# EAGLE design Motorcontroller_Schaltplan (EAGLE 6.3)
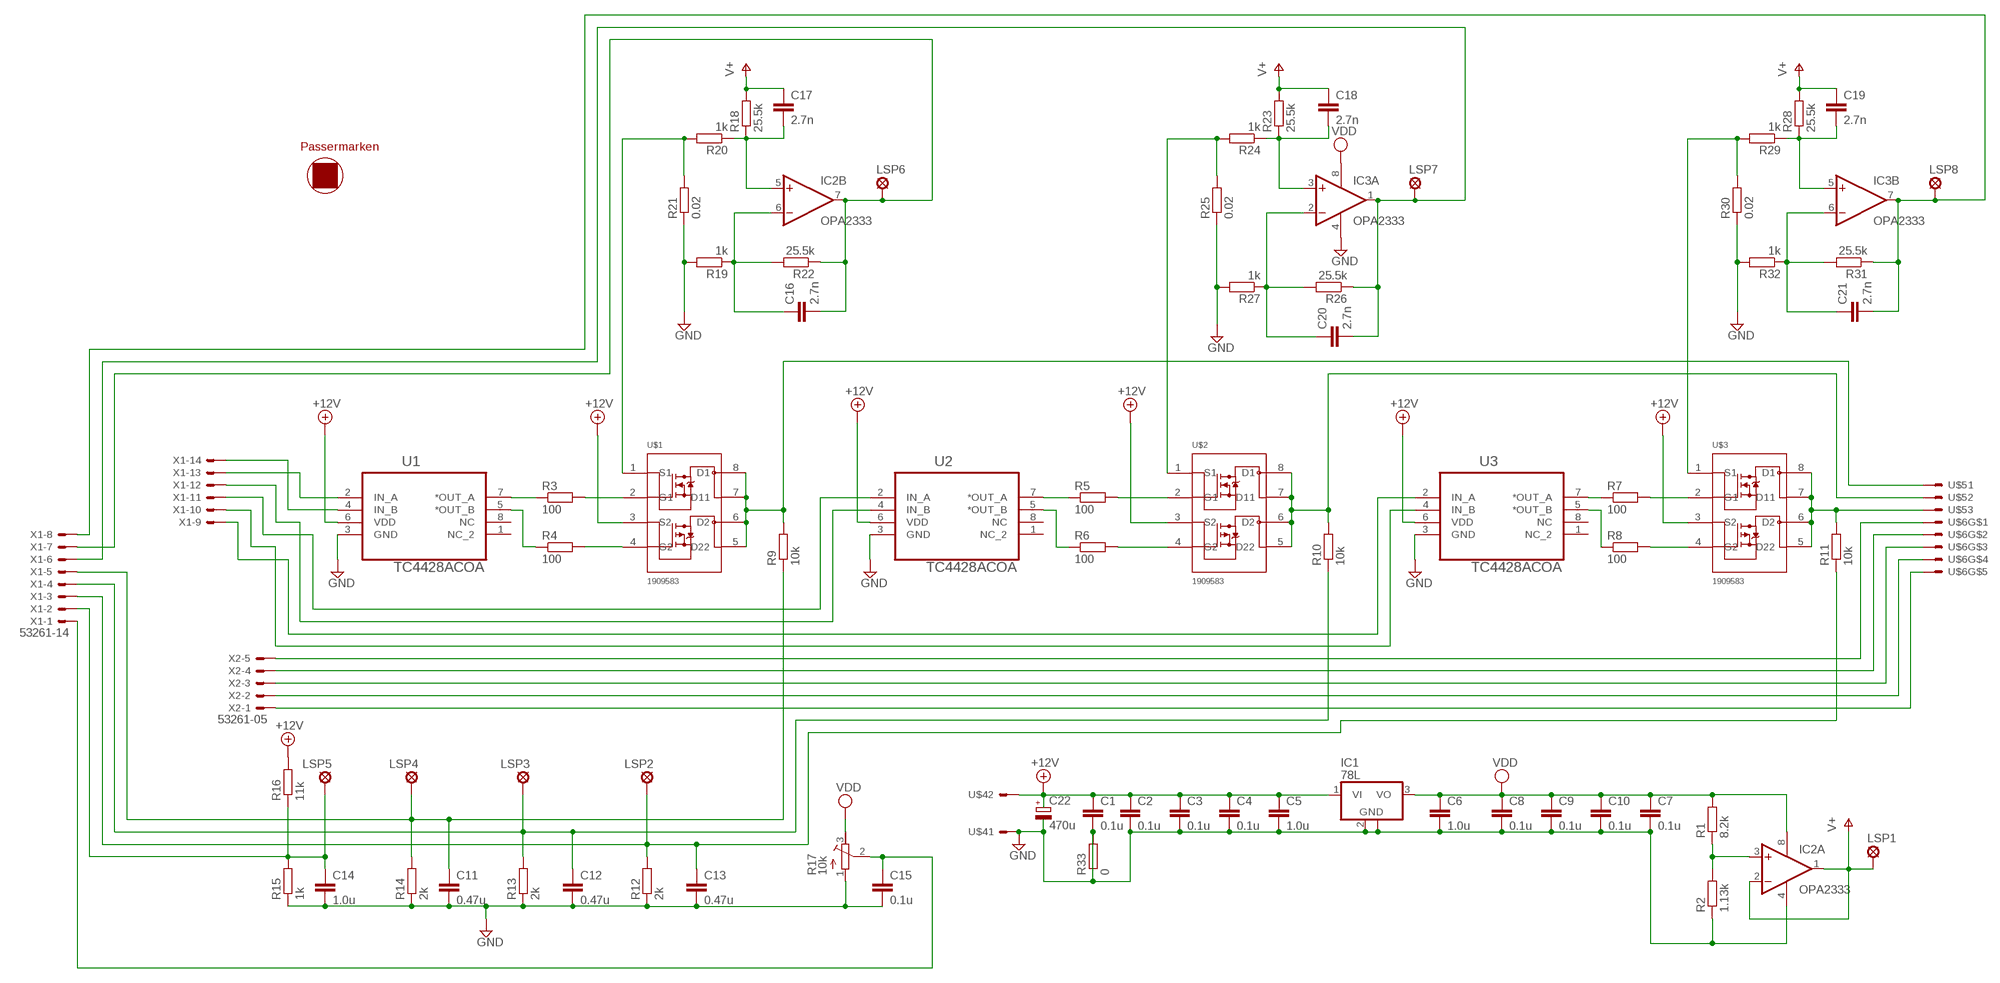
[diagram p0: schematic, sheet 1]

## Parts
C1  0.1u  C-EUC0603  [C0603]
C2  0.1u  C-EUC0603  [C0603]
C3  0.1u  C-EUC0603  [C0603]
C4  0.1u  C-EUC0603  [C0603]
C5  1.0u  C-EUC0603  [C0603]
C6  1.0u  C-EUC0603  [C0603]
C7  0.1u  C-EUC0603  [C0603]
C8  0.1u  C-EUC0603  [C0603]
C9  0.1u  C-EUC0603  [C0603]
C10  0.1u  C-EUC0603  [C0603]
C11  0.47u  C-EUC0603  [C0603]
C12  0.47u  C-EUC0603  [C0603]
C13  0.47u  C-EUC0603  [C0603]
C14  1.0u  C-EUC0603  [C0603]
C15  0.1u  C-EUC0603  [C0603]
C16  2.7n  C-EUC0603  [C0603]
C17  2.7n  C-EUC0603  [C0603]
C18  2.7n  C-EUC0603  [C0603]
C19  2.7n  C-EUC0603  [C0603]
C20  2.7n  C-EUC0603  [C0603]
C21  2.7n  C-EUC0603  [C0603]
C22  470u  CPOL-EU150CLZ-1010  [150CLZ-1010]
IC1  78L  [SOT223]
IC2  OPA2333  [SOIC8]
IC3  OPA2333  [SOIC8]
LSP1  MCS10B  [MCS10B]
LSP2  MCS10B  [MCS10B]
LSP3  MCS10B  [MCS10B]
LSP4  MCS10B  [MCS10B]
LSP5  MCS10B  [MCS10B]
LSP6  MCS10B  [MCS10B]
LSP7  MCS10B  [MCS10B]
LSP8  MCS10B  [MCS10B]
R1  8.2k  R-EU_R0603  [R0603]
R2  1.13k  R-EU_R0603  [R0603]
R3  100  R-EU_R0603  [R0603]
R4  100  R-EU_R0603  [R0603]
R5  100  R-EU_R0603  [R0603]
R6  100  R-EU_R0603  [R0603]
R7  100  R-EU_R0603  [R0603]
R8  100  R-EU_R0603  [R0603]
R9  10k  R-EU_R0603  [R0603]
R10  10k  R-EU_R0603  [R0603]
R11  10k  R-EU_R0603  [R0603]
R12  2k  R-EU_R0603  [R0603]
R13  2k  R-EU_R0603  [R0603]
R14  2k  R-EU_R0603  [R0603]
R15  1k  R-EU_R0603  [R0603]
R16  11k  R-EU_R0603  [R0603]
R17  10k  R-TRIMM  [TRIMMER3150]
R18  25.5k  R-EU_R0603  [R0603]
R19  1k  R-EU_R0603  [R0603]
R20  1k  R-EU_R0603  [R0603]
R21  0.02  R-EU_R1206  [R1206]
R22  25.5k  R-EU_R0603  [R0603]
R23  25.5k  R-EU_R0603  [R0603]
R24  1k  R-EU_R0603  [R0603]
R25  0.02  R-EU_R1206  [R1206]
R26  25.5k  R-EU_R0603  [R0603]
R27  1k  R-EU_R0603  [R0603]
R28  25.5k  R-EU_R0603  [R0603]
R29  1k  R-EU_R0603  [R0603]
R30  0.02  R-EU_R1206  [R1206]
R31  25.5k  R-EU_R0603  [R0603]
R32  1k  R-EU_R0603  [R0603]
R33  0  R-EU_R2010  [R2010]
U1  TC4428ACOA  [SOIC127P600X175-8N]
U2  TC4428ACOA  [SOIC127P600X175-8N]
U3  TC4428ACOA  [SOIC127P600X175-8N]
U$1  1909583  [SO8]
U$2  1909583  [SO8]
U$3  1909583  [SO8]
U$4  PTSM0.5/3-2.5-HSMDR44  [PTSM0,5/2-2,5-HSMDR44]
U$5  PTSM0.5/3-2.5-HSMDR44  [PTSM0,5/3-2,5-HSMDR44]
U$6  PTSM0.5/5-2.5-HSMDR44  [PTSM0,5/5-2,5-HSMDR44]
U$7  PASSERMARKEN  [MASTERSUBSTRAT-MITPASSERMARKEN]
X1  53261-14  [53261-14]
X2  53261-05  [53261-05]

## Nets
+12V: C1.1 C2.1 C3.1 C4.1 C5.1 C22.+ IC1.1(VI) R16.2 U1.6(VDD) U2.6(VDD) U3.6(VDD) U$1.3(S2) U$2.3(S2) U$3.3(S2) U$4.2
GND: C1.2 C2.2 C3.2 C4.2 C5.2 C6.2 C7.2 C8.2 C9.2 C10.2 C11.2 C12.2 C13.2 C14.2 C15.2 C22.- IC1.2(GND) IC1.4(GND) IC2.4(P:V-) IC3.4(P:V-) R2.1 R12.1 R13.1 R14.1 R15.1 R17.1 R19.2 R21.1 R25.1 R27.2 R30.1 R32.2 R33.1 R33.2 U1.3(GND) U2.3(GND) U3.3(GND) U$4.1
N$1: U1.4(IN_B) X1.14
N$2: IC2.3(A:+IN) R1.1 R2.2
N$3: U1.2(IN_A) X1.13
N$4: R3.1 U1.7(*OUT_A)
N$5: R3.2 U$1.2(G1)
N$6: R4.1 U1.5(*OUT_B)
N$7: R4.2 U$1.4(G2)
N$8: R9.2 U$1.5(D22) U$1.6(D2) U$1.7(D11) U$1.8(D1) U$5.1
N$9: U$6.1 X2.5
N$11: U2.4(IN_B) X1.12
N$12: R5.1 U2.7(*OUT_A)
N$13: R6.1 U2.5(*OUT_B)
N$14: R5.2 U$2.2(G1)
N$15: R6.2 U$2.4(G2)
N$16: R10.2 U$2.5(D22) U$2.6(D2) U$2.7(D11) U$2.8(D1) U$5.2
N$17: U2.2(IN_A) X1.11
N$18: U3.4(IN_B) X1.10
N$19: R7.1 U3.7(*OUT_A)
N$20: R7.2 U$3.2(G1)
N$21: R8.1 U3.5(*OUT_B)
N$22: R8.2 U$3.4(G2)
N$23: R11.2 U$3.5(D22) U$3.6(D2) U$3.7(D11) U$3.8(D1) U$5.3
N$24: U$6.2 X2.4
N$25: C13.1 LSP2.MP R11.1 R12.2 X1.3
N$26: U3.2(IN_A) X1.9
N$28: C11.1 LSP4.MP R9.1 R14.2 X1.5
N$29: C12.1 LSP3.MP R10.1 R13.2 X1.4
N$31: C14.1 LSP5.MP R15.2 R16.1 X1.2
N$32: C15.1 R17.2 X1.1
N$33: C18.2 IC3.3(A:+IN) R23.1 R24.1
N$34: C17.2 IC2.5(B:+IN) R18.1 R20.1
N$35: R20.2 R21.2 U$1.1(S1)
N$36: R24.2 R25.2 U$2.1(S1)
N$37: C16.1 IC2.6(B:-IN) R19.1 R22.2
N$38: C16.2 IC2.7(B:OUT) LSP6.MP R22.1 X1.7
N$39: C20.1 IC3.2(A:-IN) R26.2 R27.1
N$40: C20.2 IC3.1(A:OUT) LSP7.MP R26.1 X1.6
N$41: C19.2 IC3.5(B:+IN) R28.1 R29.1
N$42: R29.2 R30.2 U$3.1(S1)
N$43: C21.1 IC3.6(B:-IN) R31.2 R32.1
N$44: C21.2 IC3.7(B:OUT) LSP8.MP R31.1 X1.8
N$47: U$6.3 X2.3
N$48: U$6.4 X2.2
N$49: U$6.5 X2.1
V+: C17.1 C18.1 C19.1 IC2.1(A:OUT) IC2.2(A:-IN) LSP1.MP R18.2 R23.2 R28.2
VDD: C6.1 C7.1 C8.1 C9.1 C10.1 IC1.3(VO) IC2.8(P:V+) IC3.8(P:V+) R1.2 R17.3
Unconnected: U1.1(NC_2) U1.8(NC) U2.1(NC_2) U2.8(NC) U3.1(NC_2) U3.8(NC)

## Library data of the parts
C1-C21 = rcl:C-EU: CAPACITOR, European symbol
C22 = rcl:CPOL-EU: POLARIZED CAPACITOR, European symbol
IC1 = BLDC:78L*: POSITOIV-VOLTAGE REGULATORS Output up to 100 mA Source: http://focus.ti.com/lit/ds/symlink/ua78l05.pdf
IC2 IC3 = BLDC:OPA2333: DUAL 1.8V, microPOWER CMOS OPERATIONAL AMPLIFIERS Zerø-Drift Series Source: Texas Instruments (Burr-Brown) .. U11 opa333 Operational Amp.pdf
LSP1-LSP8 = solpad:MCS10B: SOLDER PAD
R1-R16 R18-R33 = rcl:R-EU_: RESISTOR, European symbol
R17 = BLDC:R-TRIMM: Trimm resistor
U1-U3 = TC4428COA:TC4428ACOA: DRIVER, MOSFET, DUAL 1.5A; MPN: TC4428ACOA; OC_FARNELL: 1332312; OC_NEWARK: 34M8781; PACKAGE: SOIC-8; SUPPLIER: Microchip
U$1-U$3 = BLDC:1909583
U$4 = Phoenix_SMD:PTSM0.5/3-2.5-HSMDR44
U$5 = Phoenix_SMD (2):PTSM0.5/3-2.5-HSMDR44
U$6 = Phoenix_SMD (2):PTSM0.5/5-2.5-HSMDR44
U$7 = lmhs:PASSERMARKEN
X1 = con-molex:53?-14: CONNECTOR wire to board 1.25 mm (.049 inch) pitch header; OC_FARNELL: 1125364; OC_NEWARK: unknown
X2 = con-molex:53?-05: CONNECTOR wire to board 1.25 mm (.049 inch) pitch header; OC_FARNELL: 1433644; OC_NEWARK: unknown

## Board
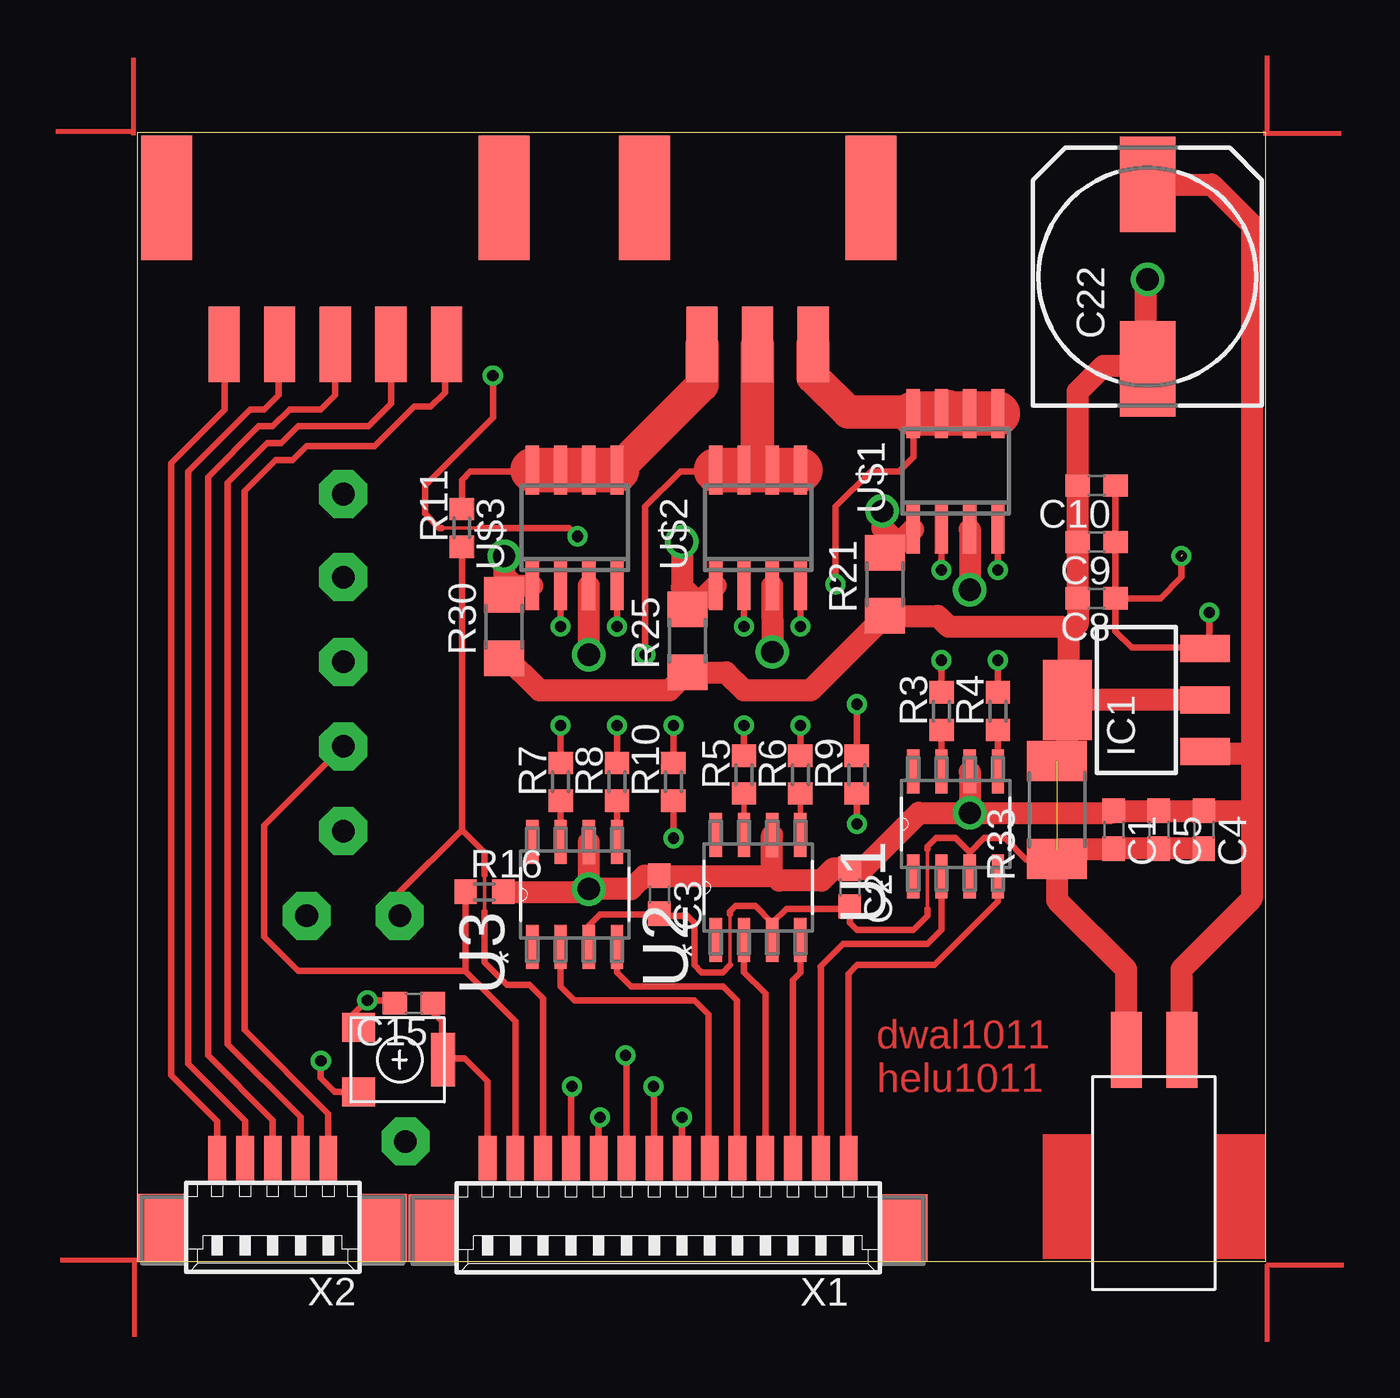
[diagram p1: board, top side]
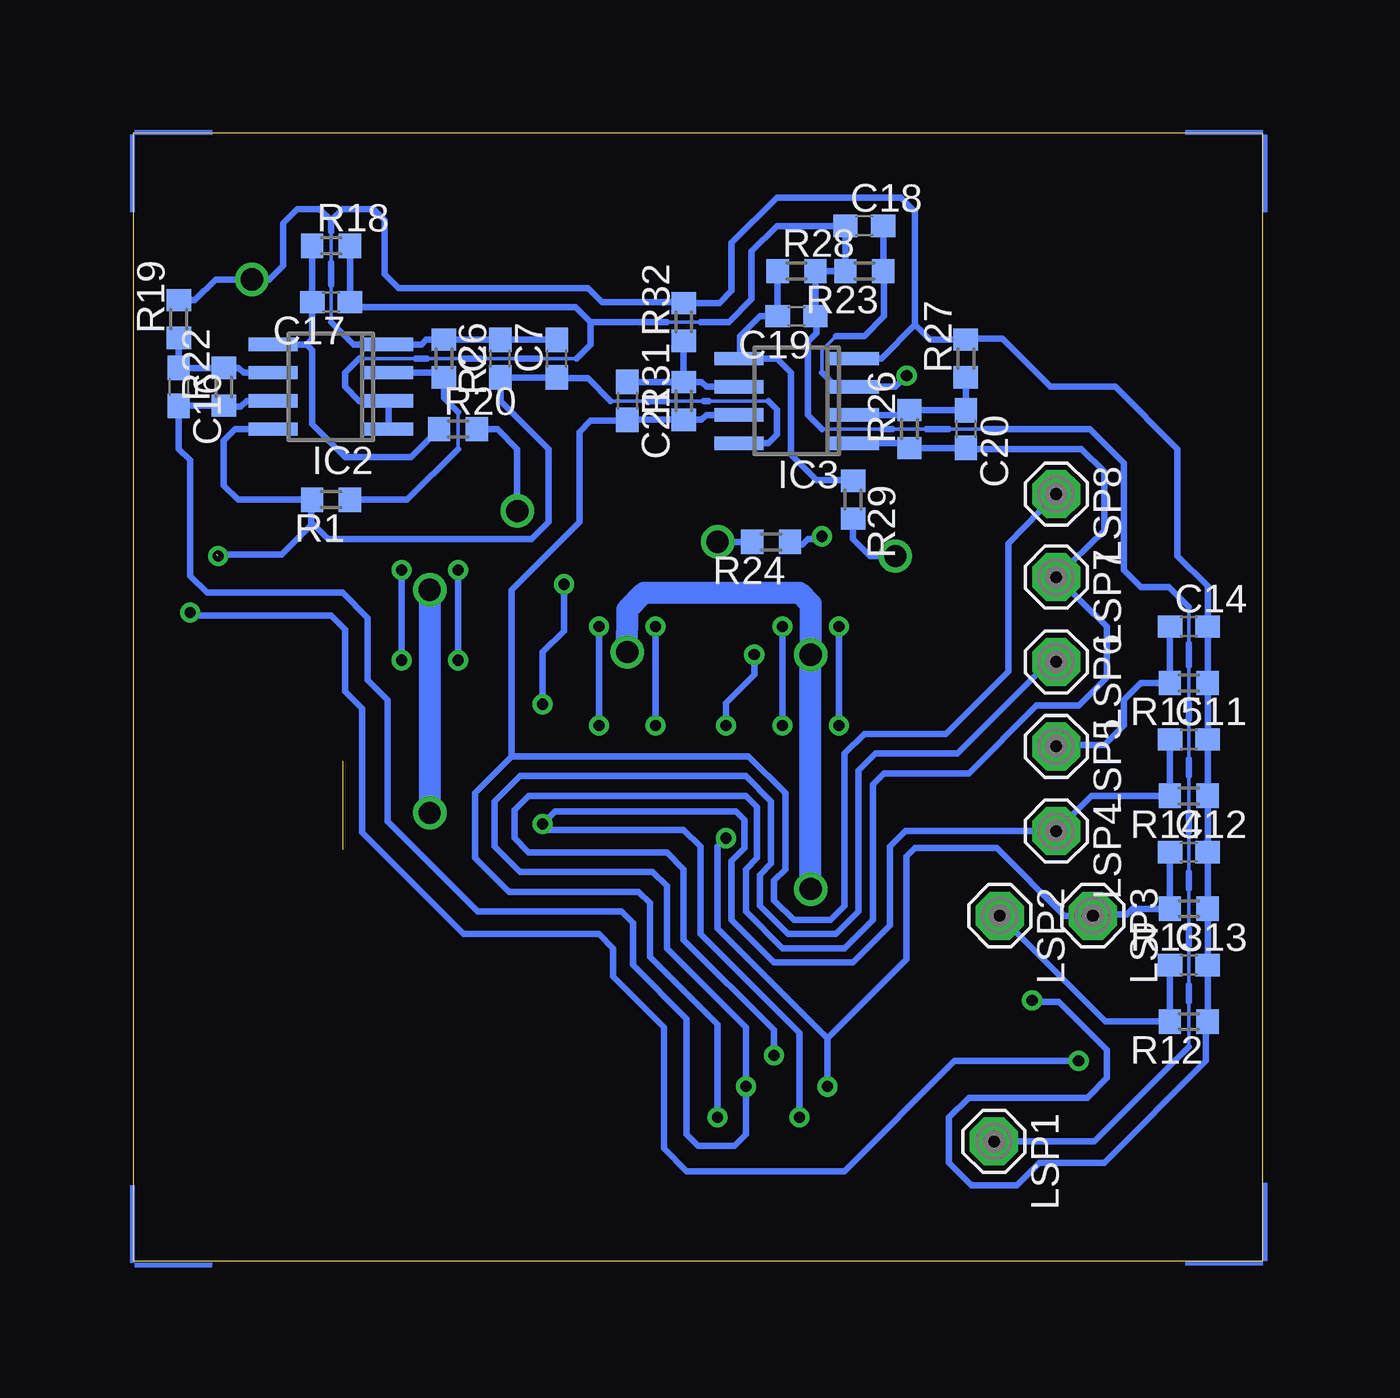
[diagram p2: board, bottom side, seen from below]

Size 50.8 x 50.8 mm. Coordinates in mm from the lower left corner, seen from the top.
Outline: 0,0 50.8,0 50.8,50.8 0,50.8 0,0
Copper layers (1*16): Top 0.035mm / dielectric 1.5mm / Bottom 0.035mm
Design rules "default *": minimum track width 0.15mm, minimum drill 24mil, track to track 0.2mm, track to pad 0.2mm, pad to pad 0.2mm, via to via 0.2mm, smd to smd 0.15mm, copper to edge 40mil, drill to drill 8mil, minimum pad ring 10mil, minimum via ring 8mil, stop-mask expansion 4mil, vias tented up to drill 0mil, thermal gap 10mil

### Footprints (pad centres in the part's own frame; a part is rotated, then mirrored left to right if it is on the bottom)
C0603 = smd 1.1 x 1: 1 -0.85,0; 2 0.85,0
150CLZ-1010 = smd 4.3 x 2.5: + 4.15,0; - -4.15,0
SOT223 = smd 1.219 x 2.235: 1 -2.311,-3.099; 2 0,-3.099; 3 2.311,-3.099 | smd 3.6 x 2.2: 4 0,3.099
SOIC8 = smd 0.6 x 2.2: 1 0,-0.06; 2 1.27,-0.06; 3 2.54,-0.06; 4 3.81,-0.06; 5 3.81,5.14; 6 2.54,5.14; 7 1.27,5.14; 8 0,5.14
MCS10B = drill 1.016 pad 2.159 octagon: MP 0,0
R0603 = smd 1 x 1.1: 1 -0.85,0; 2 0.85,0
TRIMMER3150 = smd 1.3 x 1.5: 1 -1.45,-1.85; 3 1.45,-1.85 | smd 2.4 x 1.1: 2 0,1.95
R1206 = smd 1.6 x 1.803: 1 -1.422,0; 2 1.422,0
R2010 = smd 1.8 x 2.7: 1 -2.2,0; 2 2.2,0
SOIC127P600X175-8N = smd 1.981 x 0.559: 1 -2.362,1.905; 2 -2.362,0.635; 3 -2.362,-0.635; 4 -2.362,-1.905; 5 2.362,-1.905; 6 2.362,-0.635; 7 2.362,0.635; 8 2.362,1.905
SO8 = smd 0.6 x 2.2: 1 0,-0.06; 2 1.27,-0.06; 3 2.54,-0.06; 4 3.81,-0.06; 5 3.81,5.14; 6 2.54,5.14; 7 1.27,5.14; 8 0,5.14
PTSM0,5/2-2,5-HSMDR44 = smd 1.4 x 3.4: 1 2.6,6.6; 2 5.1,6.6
PTSM0,5/3-2,5-HSMDR44 = smd 1.4 x 3.4: 1 2.6,6.6; 2 5.1,6.6; 3 7.6,6.6 | smd 2.3 x 5.6: P$1 0,0; P$2 10.2,0
PTSM0,5/5-2,5-HSMDR44 = smd 1.4 x 3.4: 1 2.6,6.6; 2 5.1,6.6; 3 7.6,6.6; 4 10.1,6.6; 5 12.6,6.6 | smd 2.3 x 5.6: P$1 0,0; P$8 15.2,0
53261-14 = smd 0.8 x 2: 1 8.125,-2.5; 2 6.875,-2.5; 3 5.625,-2.5; 4 4.375,-2.5; 5 3.125,-2.5; 6 1.875,-2.5; 7 0.625,-2.5; 8 -0.625,-2.5; 9 -1.875,-2.5; 10 -3.125,-2.5; 11 -4.375,-2.5; 12 -5.625,-2.5; 13 -6.875,-2.5; 14 -8.125,-2.5 | smd 2.1 x 3: S1 10.625,0.625; S2 -10.625,0.625
53261-05 = smd 0.8 x 2: 1 2.5,-2.5; 2 1.25,-2.5; 3 0,-2.5; 4 -1.25,-2.5; 5 -2.5,-2.5 | smd 2.1 x 3: S1 5,0.625; S2 -5,0.625

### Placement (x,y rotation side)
C1  43.94,19.43 270 top
C2  32.07,16.83 270 top
C3  23.5,16.51 270 top
C4  48.01,19.43 270 top
C5  45.97,19.43 270 top
C6  34.29,40.64 90 bottom
C7  31.75,40.64 90 bottom
C8  43.18,29.84 180 top
C9  43.18,32.38 180 top
C10  43.18,34.92 180 top
C11  3.3,23.5 0 bottom
C12  3.3,18.41 0 bottom
C13  3.3,13.34 0 bottom
C14  3.3,28.57 0 bottom
C15  12.45,11.62 180 top
C16  48.77,39.37 270 bottom
C17  41.91,43.18 180 bottom
C18  17.91,46.61 0 bottom
C19  20.95,42.55 180 bottom
C20  13.34,37.47 270 bottom
C21  28.57,38.73 270 bottom
C22  45.47,44.32 90 top
IC1  44.96,25.27 90 top
IC2  39.37,37.47 90 bottom
IC3  18.41,36.83 90 bottom
LSP1  12.07,5.4 270 bottom
LSP2  11.81,15.56 270 bottom
LSP3  7.62,15.56 270 bottom
LSP4  9.27,19.37 270 bottom
LSP5  9.27,23.18 270 bottom
LSP6  9.27,26.99 270 bottom
LSP7  9.27,30.8 270 bottom
LSP8  9.27,34.54 270 bottom
R1  41.91,34.29 180 bottom
R2  36.83,40.64 270 bottom
R3  36.2,24.77 90 top
R4  38.73,24.77 90 top
R5  27.3,21.91 90 top
R6  29.84,21.91 90 top
R7  19.05,21.59 90 top
R8  21.59,21.59 90 top
R9  32.38,21.91 90 top
R10  24.13,21.59 90 top
R11  14.61,33.02 90 top
R12  3.3,10.79 180 bottom
R13  3.3,15.88 180 bottom
R14  3.3,20.95 180 bottom
R15  3.3,26.04 180 bottom
R16  15.62,16.64 0 top
R17  11.81,9.08 270 top
R18  41.91,45.72 0 bottom
R19  48.77,42.42 90 bottom
R20  36.2,37.47 0 bottom
R21  33.66,30.48 90 top
R22  46.74,39.37 90 bottom
R23  17.91,44.58 180 bottom
R24  22.1,32.38 180 bottom
R25  24.77,27.94 90 top
R26  15.88,37.47 90 bottom
R27  13.34,40.64 90 bottom
R28  20.95,44.58 0 bottom
R29  18.41,34.29 270 bottom
R30  16.51,28.57 90 top
R31  26.04,38.73 90 bottom
R32  26.04,42.29 90 bottom
R33  41.4,20.32 90 top
U1  36.83,19.68 90 top
U2  27.94,16.83 90 top
U3  19.68,16.51 90 top
U$1  34.92,33.02 0 top
U$2  26.04,30.48 0 top
U$3  17.78,30.48 0 top
U$4  41.91,2.92 0 top
U$5  33.02,47.88 180 top
U$6  16.51,47.88 180 top
U$7  not placed on the board
X1  23.89,2.14 180 top
X2  6.1,2.16 180 top

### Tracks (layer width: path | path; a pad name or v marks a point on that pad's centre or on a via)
+12V  (via drill 1)
  Top 1: IC1.1 48.16,22.86 50.16,22.86 | U$4.2 47.01,13.16 50.16,16.32 50.16,20.32 | C22.+ 48.36,48.47 50.16,46.67 50.16,22.86 | 50.16,22.86 50.16,20.32 | 50.16,20.32 50.13,20.28 C4.1 C5.1 C1.1 43.85,20.19 v37.47,20.19 | 32.17,17.78 C2.1 | C2.1 31.33,17.68 30.8,17.14 28.89,17.14 28.57,17.46 | 28.57,17.46 U2.6 | 28.57,17.46 28.47,17.36 C3.1 22.82,17.36 22.23,16.76 v20.32,16.76 | U$1.3 v37.47,30.23 | v20.32,27.31 U$3.3 | v20.32,16.76 U3.6 | R16.2 20.19,16.64 v20.32,16.76 | U$2.3 v28.58,27.43 | U1.6 v37.47,20.19 | v37.47,20.19 35.18,20.19 32.64,17.65 32.09,17.65 C2.1
  Bottom 1: v37.47,30.23 v37.47,20.19 | v20.32,16.76 v20.32,27.31 20.32,29.59 20.83,30.1 27.81,30.1 28.57,29.34 v28.58,27.43
GND  (via drill 0.5, 1)  (1 unrouted)
  Top 0.15: 40.72,18.12 R33.1 | 26.67,15.62 26.67,13.34 | 35.56,18.54 35.56,15.88
  Top 0.254: 20.32,13.34 U3.3
  Top 0.3: U1.3 37.47,18.41 | 37.47,18.41 38.1,19.05 39.05,19.05 40.01,18.1 40.7,18.1 40.72,18.12 | 37.47,18.41 36.83,19.05 35.94,19.05 35.56,18.67 35.56,18.54 | 35.56,15.88 35.56,15.56 34.92,14.92 32.38,14.92 32.07,15.24 32.07,15.88 | 32.07,15.88 C2.2 | 32.07,15.88 29.21,15.88 28.57,15.24 | U2.3 28.57,15.24 | 28.57,15.24 27.81,16 26.92,16 26.67,15.75 26.67,15.62 | 26.67,13.34 26.35,13.02 25.4,13.02 25.08,13.34 25.08,15.24 24.77,15.56 23.6,15.56 C3.2 23.46,15.62 20.83,15.62 20.32,15.11 U3.3 | R17.1 9.65,10.53 9.65,11.05 v10.35,11.75 11.3,11.75 11.43,11.62 C15.2
  Top 1: R30.1 16.51,27.3 18.1,25.72 23.96,25.72 R25.1 | 24.77,26.67 R25.1 | IC1.2 IC1.4 | C4.2 C5.2 C1.2 43.9,18.54 41.4,18.54 R33.1 41.4,16.26 44.51,13.15 U$4.1 | R33.2 41.86,22.98 IC1.4 | 45.32,40.32 43.5,40.32 42.33,39.16 C10.2 C9.2 C8.2 42.33,28.68 41.91,28.26 | 45.32,40.32 C22.- | 41.91,28.26 41.91,25.32 IC1.4 | 41.91,28.26 41.59,28.57 36.51,28.57 36.03,29.06 R21.1 30.31,25.72 27.3,25.72 26.5,26.52 R25.1 | 45.32,40.32 45.4,40.32 45.4,44.13 v45.47,44.2
  Bottom 0.15: R27.2 13.12,41.49 | 15.03,41.49 15.03,41.57 | 26.07,43.18 R32.2 | 41.91,42.29 41.91,43.94 | 41.91,44.96 41.91,46.35
  Bottom 0.3: R19.2 48.05,43.27 47.12,44.2 v45.47,44.2 44.7,44.2 44.07,44.83 44.07,46.74 43.43,47.37 42.42,47.37 41.91,46.86 | 41.91,46.86 41.4,47.37 40.01,47.37 39.5,46.86 39.5,44.45 38.86,43.81 30.35,43.81 29.72,43.18 26.07,43.18 | 41.91,42.29 40.89,41.27 IC2.4 37.85,41.27 37.63,41.49 R2.1 C6.2 C7.2 | 41.91,43.94 41.91,44.96 | 41.91,46.35 41.91,46.86 | R32.2 24.42,43.14 23.88,43.69 23.88,45.85 21.84,47.88 16.26,47.88 15.62,47.24 15.62,42.16 | 15.62,42.16 15.03,41.57 14.95,41.49 R27.2 13.3,41.53 11.68,41.53 9.53,39.37 6.6,39.37 3.81,36.58 3.81,31.75 2.45,30.39 C14.2 R15.1 C11.2 R14.1 C12.2 R13.1 C13.2 R12.1 2.54,10.71 2.54,9.02 7.11,4.45 10.03,4.45 11.05,3.43 13.08,3.43 14.1,4.45 14.1,6.48 13.21,7.37 7.87,7.37 6.99,8.26 6.99,9.53 9.14,11.68 10.29,11.68 v10.35,11.75 | IC3.4 17.14,40.64 15.62,42.16
N$1
  Top 0.3: X1.14 32,4.66 32,12.95 32.38,13.34 35.88,13.34 38.73,16.19 U1.4
N$2
  Bottom 0.15: R2.2 37.05,40.01 | 36.2,36.58 36.2,38.23
  Bottom 0.3: R1.1 38.48,34.29 36.2,36.58 | 36.2,38.23 36.83,38.86 R2.2 | 37.05,40.01 IC2.3
N$3
  Top 0.3: U1.2 36.2,14.92 35.56,14.29 31.75,14.29 30.75,13.29 30.77,13.27 X1.13
N$4
  Top 0.3: R3.1 U1.7
N$5  (via drill 0.5)
  Top 0.3: v36.2,31.12 U$1.2 | v36.2,27.06 R3.2
  Bottom 0.3: v36.2,31.12 v36.2,27.06
N$6
  Top 0.3: R4.1 U1.5
N$7  (via drill 0.5)
  Top 0.3: U$1.4 v38.74,31.12 | v38.74,27.06 R4.2
  Bottom 0.3: v38.74,31.12 v38.74,27.06
N$8  (via drill 0.5)
  Top 0.3: 34.87,38.1 U$1.8 34.92,36.2 34.29,35.56 33.02,35.56 31.43,33.97 v31.43,30.48 | R9.2 v32.39,25.08
  Top 1.5: 36.52,38.48 U$1.7 | U$5.1 30.42,39.81 32,38.23 34.86,38.23 U$1.8
  Top 2: U$1.5 U$1.6 U$1.7 U$1.8
  Bottom 0.3: v31.43,30.48 31.43,28.38 32.38,27.43 v32.39,25.08
N$9
  Top 0.3: X2.5 8.6,6.64 4.83,10.41 4.83,34.67 6.22,36.07 6.99,36.07 7.62,36.7 10.67,36.7 12.45,38.48 13.21,38.48 13.84,39.12 13.84,41.21 U$6.1
N$11
  Top 0.3: U2.4 29.84,13.02 29.5,12.67 29.52,12.66 X1.12
N$12
  Top 0.254: U2.7 R5.1
N$13
  Top 0.254: U2.5 R6.1
N$14  (via drill 0.5)
  Top 0.3: U$2.2 v27.31,28.58 | R5.2 v27.31,24.13
  Bottom 0.3: v27.31,28.58 v27.31,24.13
N$15  (via drill 0.5)
  Top 0.3: U$2.4 v29.85,28.58 | R6.2 v29.85,24.13
  Bottom 0.3: v29.85,28.58 v29.85,24.13
N$16  (via drill 0.5)
  Top 0.3: v22.86,27.31 22.86,33.97 24.45,35.56 25.98,35.56 U$2.8 | R10.2 v24.13,24.13
  Top 1.5: U$2.5 28,35.62 27.94,35.56 28.3,35.56 | U$5.2 27.92,35.64 27.94,35.62
  Top 2: U$2.8 U$2.7 27.94,35.62 U$2.6 U$2.5
  Bottom 0.3: v22.86,27.31 22.86,26.42 24.13,25.15 v24.13,24.13
N$17
  Top 0.3: U2.2 27.3,13.02 28.27,12.06 X1.11
N$18
  Top 0.3: U3.4 21.59,13.02 22.23,12.38 26.35,12.38 26.99,11.75 26.99,4.67 X1.10
N$19
  Top 0.3: U3.7 R7.1
N$20  (via drill 0.5)
  Top 0.3: v19.05,28.58 U$3.2 | R7.2 v19.05,24.13
  Bottom 0.3: v19.05,24.13 v19.05,28.58
N$21
  Top 0.3: U3.5 R8.1
N$22  (via drill 0.5)
  Top 0.3: v21.59,28.58 U$3.4 | R8.2 v21.59,24.13
  Bottom 0.3: v21.59,24.13 v21.59,28.58
N$23
  Top 0.3: R11.2 14.61,35.18 14.99,35.56 17.72,35.56 U$3.8
  Top 1.5: U$3.6 20.38,35.62 | U$5.3 25.42,39.45 U$3.5
  Top 2: U$3.8 U$3.7 U$3.6 U$3.5
N$24
  Top 0.3: X2.4 7.35,6.5 4.06,9.78 4.06,35.05 5.84,36.83 6.48,36.83 7.24,37.59 10.41,37.59 11.43,38.61 11.43,41.26 U$6.2
N$25
  Top 0.15: 15.62,15.75 15.62,17.4
  Top 0.3: X1.3 18.27,11.83 17.65,12.45 16.64,12.45 15.62,13.46 15.62,15.75 | R11.1 14.61,19.43 | 15.62,17.4 15.62,18.41 14.61,19.43 | LSP2.MP 11.81,16.64 14.61,19.43
  Bottom 0.3: C13.1 R12.2 7.05,10.79 LSP2.MP
N$26
  Top 0.3: U3.2 19.05,12.38 19.68,11.75 25.08,11.75 25.72,11.11 25.72,4.69 X1.9
N$28  (via drill 0.5)
  Top 0.3: v32.39,19.69 R9.1 | X1.5 20.77,6.42 v20.83,6.48
  Bottom 0.15: R14.2 4.45,20.95
  Bottom 0.3: C11.1 R14.2 | 4.45,20.95 7.68,20.95 LSP4.MP 16.06,19.37 16.76,18.67 16.76,15.11 18.41,13.46 21.97,13.46 23.88,15.37 23.88,18.03 23.3,18.61 23.3,19.88 23.69,20.26 31.82,20.26 v32.39,19.69 32.13,19.43 26.04,19.43 25.27,18.67 25.27,14.73 20.83,10.29 v20.83,6.48
N$29  (via drill 0.5)
  Top 0.3: v24.13,19.05 R10.1 | X1.4 19.52,7.83 v19.56,7.87
  Bottom 0.3: C12.1 R13.2 5.84,15.88 6.1,15.62 7.56,15.62 LSP3.MP 8.83,15.56 8.89,15.56 11.94,18.61 15.62,18.61 16,18.22 16,13.59 19.56,10.04 | v24.13,19.05 24.51,18.67 24.51,14.99 19.56,10.04 | v19.56,7.87 19.56,10.04
N$31
  Top 0.3: X1.2 17.02,10.8 14.77,13.04 | R16.1 14.77,13.04 | 14.77,13.04 14.73,13.08 7.24,13.08 5.71,14.61 5.71,19.62 LSP5.MP
  Bottom 0.3: C14.1 R15.2 5.46,26.04 6.22,25.27 6.22,24.13 7.11,23.24 9.21,23.24 LSP5.MP
N$32
  Top 0.3: X1.1 15.77,8.11 14.73,9.14 13.82,9.14 R17.2 13.72,9.13 13.72,10.79 13.3,11.21 C15.1
N$33  (via drill 0.5)
  Top 0.15: 13.72,33.02 15.37,33.02
  Top 0.3: v16,39.88 16,37.97 12.95,34.92 12.95,33.66 13.59,33.02 13.72,33.02 | 15.37,33.02 19.43,33.02 v19.81,32.64
  Bottom 0.15: IC3.3 19.05,39.37 | 17.02,44.23 R23.1 | 19.81,40.01 19.81,41.02 19.18,41.66
  Bottom 0.3: C18.2 R23.1 17.02,44.54 17.02,42.55 17.91,41.66 19.18,41.66 | 19.81,40.01 19.18,39.37 19.05,39.37 16.51,39.37 v16,39.88 | R24.1 21.12,32.26 20.7,32.26 20.45,32.51 19.94,32.51 v19.81,32.64
N$34
  Bottom 0.15: IC2.5 44.45,41.34
  Bottom 0.3: R20.1 38.31,36.2 41.27,36.2 42.76,37.68 42.76,41.02 43.01,41.27 | R18.1 C17.2 42.76,41.53 43.01,41.27 | IC2.5 43.01,41.27
N$35  (via drill 1)
  Top 0.3: U$1.1 34.61,32.96 34.1,32.45 33.78,32.13 33.78,32
  Top 1: U$1.1 33.87,31.9 R21.2 33.53,32.03 | v33.53,33.78 33.53,33.02 34.1,32.45
  Bottom 0.3: v33.53,33.78 33.53,36.58 34.42,37.47 R20.2
N$36  (via drill 1)
  Top 1: R25.2 24.98,29.36 25.24,29.62 | 25.24,29.62 U$2.1 | v24.51,32.39 24.51,30.35 25.24,29.62
  Bottom 0.3: R24.2 v24.51,32.39
N$37
  Bottom 0.15: IC2.6 44.73,40.22
  Bottom 0.3: IC2.6 45.85,40.01 46.06,40.22 R22.2 C16.1 R19.1
N$38  (via drill 0.5)
  Top 0.3: X1.7 23.27,7.85 v23.24,7.87
  Bottom 0.15: IC2.7 44.73,38.52
  Bottom 0.3: LSP6.MP 9.59,26.99 13.72,22.86 17.4,22.86 18.16,22.1 18.16,15.75 19.18,14.73 21.34,14.73 22.61,16 22.61,17.4 22.1,17.91 22.1,20.7 23.24,21.84 33.4,21.84 34.54,20.7 34.54,18.67 33.4,17.53 27.43,17.53 26.8,16.89 26.8,14.1 23.24,10.54 v23.24,7.87 23.24,5.71 23.75,5.21 25.4,5.21 25.91,5.71 25.91,10.92 28.32,13.34 28.32,15.24 28.83,15.75 35.31,15.75 39.37,19.81 39.37,25.27 40.26,26.16 40.26,28.96 41.4,30.1 47.5,30.1 48.26,30.86 48.26,36.07 48.77,36.58 C16.2 R22.1 46.7,38.48 45.97,38.48 45.72,38.73 IC2.7
N$39
  Bottom 0.15: 16.09,38.1 R26.2
  Bottom 0.3: R26.2 C20.1 R27.1 | 16.09,38.1 IC3.2
N$40  (via drill 0.5)
  Top 0.3: X1.6 22.02,9.22 v21.97,9.27
  Bottom 0.15: 16.09,36.83 R26.1
  Bottom 0.3: R26.1 C20.2 13.3,36.58 8.13,36.58 7.11,35.56 7.11,32.89 LSP7.MP 6.99,28.57 6.99,26.29 8.26,25.02 10.16,25.02 13.21,21.97 17.02,21.97 17.53,21.46 17.53,15.37 18.8,14.1 21.59,14.1 23.24,15.75 23.24,17.65 22.73,18.16 22.73,20.45 23.24,20.95 33.02,20.95 33.66,20.32 33.66,19.05 33.02,18.41 26.8,18.41 26.04,17.65 26.04,14.48 21.97,10.41 v21.97,9.27 | 16.09,36.83 IC3.1
N$41
  Bottom 0.3: R28.1 C19.2 22.61,42.55 23.5,41.66 23.5,40.7 IC3.5 21.84,40.64 21.21,40.01 21.21,36.32 20.07,35.18 18.45,35.18 R29.1
N$42  (via drill 1)
  Top 0.15: R30.2 16.93,30.42 16.51,30.42
  Top 1: U$3.1 16.93,30.42 16.51,30.84 v16.51,31.75
  Bottom 0.15: R29.2 18.2,33.66
  Bottom 0.3: v16.51,31.75 17.65,31.75 18.41,32.51 R29.2
N$43
  Bottom 0.15: 23.77,39.59 IC3.6
  Bottom 0.3: R31.2 R32.1 | R31.2 C21.1 | R31.2 25.23,39.59 25.02,39.37 IC3.6
N$44  (via drill 0.5)
  Top 0.3: X1.8 v24.52,6.47 v24.51,6.48
  Bottom 0.3: 33.78,22.73 35.43,21.08 35.43,18.16 33.91,16.64 28.07,16.64 27.56,16.13 27.56,13.72 24.51,10.67 v24.51,6.48 | LSP8.MP 11.43,32.32 11.43,26.54 14.22,23.75 17.91,23.75 18.8,22.86 18.8,16 19.43,15.37 21.08,15.37 21.97,16.26 21.97,17.14 21.46,17.65 21.46,21.08 23.11,22.73 33.78,22.73 | IC3.7 25.02,38.1 25.23,37.88 R31.1 C21.2 28.61,37.85 30.23,37.85 30.73,37.34 30.73,33.27 33.78,30.23 33.78,22.73
N$47
  Top 0.3: X2.3 6.1,6.35 3.17,9.27 3.17,35.31 5.46,37.59 6.1,37.59 6.86,38.35 8.26,38.35 8.89,38.99 8.89,41.26 U$6.3
N$48
  Top 0.3: X2.2 4.85,6.33 2.29,8.89 2.29,35.56 5.08,38.35 5.71,38.35 6.35,38.99 6.35,41.22 U$6.4 6.35,41.21
N$49
  Top 0.3: X2.1 3.6,6.31 1.52,8.38 1.52,35.94 3.94,38.35 3.94,41.25 U$6.5 | U$6.5 | U$6.5
V+
  Bottom 0.15: C17.1 41.27,42.97 | 20.32,42.55 C19.1 20.32,42.33 | 40.64,40.64 38.1,40.64 | 37.59,40.64 36.07,40.64 | 35.18,40.64 33.53,40.64 | 26.8,42.29 25.27,42.29 | 30.86,40.64 32.51,40.64 | 19.81,37.47 17.14,37.47 | 16.64,37.47 15.11,37.47 | 14.1,37.47 12.45,37.47 | 3.3,29.46 3.3,27.81 | 3.3,26.8 3.3,25.15 | 3.3,24.38 3.3,22.61 | 3.3,21.84 3.3,20.07 | 3.3,19.3 3.3,17.53 | 3.3,16.76 3.3,14.99 | 3.3,14.22 3.3,12.45 | 3.3,11.68 3.3,9.65
  Bottom 0.3: LSP1.MP 7.56,5.4 3.3,9.65 | 19.81,37.47 20.45,38.1 20.45,41.4 20.07,41.78 20.07,42.51 C19.1 R28.2 R23.2 C18.1 21.84,46.61 22.99,45.47 22.99,43.31 24,42.29 25.27,42.29 | C17.1 R18.2 | IC2.1 IC2.2 40.64,38.73 41.27,39.37 41.27,40.01 40.64,40.64 | 38.1,40.64 37.59,40.64 | 36.07,40.64 35.18,40.64 | 33.53,40.64 32.51,40.64 | 30.23,42.29 30.23,41.27 30.86,40.64 | 41.27,42.97 30.9,42.97 30.23,42.29 | 30.23,42.29 26.8,42.29 | 3.3,29.46 4.19,30.35 5.46,30.35 6.22,31.11 6.22,35.94 7.75,37.47 12.45,37.47 | 17.14,37.47 16.64,37.47 | 15.11,37.47 14.1,37.47 | 3.3,27.81 3.3,26.8 | 3.3,25.15 3.3,24.38 | 3.3,22.61 3.3,21.84 | 3.3,20.07 3.3,19.3 | 3.3,17.53 3.3,16.76 | 3.3,14.99 3.3,14.22 | 3.3,12.45 3.3,11.68
VDD  (via drill 0.5)  (1 unrouted)
  Top 0.15: IC1.3 48.01,27.64
  Top 0.3: C10.1 C9.1 C8.1 | v46.99,31.75 46.99,30.8 46.04,29.84 C8.1 | 48.01,27.64 44.76,27.64 44.03,28.36 C8.1 | R17.3 8.88,7.63 8.26,8.26 v8.26,9.02 | v48.26,29.21 48.26,27.79 IC1.3
  Bottom 0.15: 42.76,34.45 42.91,34.29 R1.2 | C6.1 34.08,40.01 33.86,39.79 | 25.15,38.73 26.8,38.73 | 27.69,38.73 29.34,38.73 | 22.23,38.73 24.89,38.73
  Bottom 0.3: 47.05,31.81 44.14,31.81 42.8,33.15 42.8,33.27 | 42.8,33.27 42.8,34.25 R1.2 | 42.76,34.45 R1.2 | IC2.8 46.23,37.47 46.74,36.96 46.74,34.92 46.1,34.29 R1.2 | 33.86,39.79 C7.1 31.71,39.75 30.35,39.75 29.34,38.73 | 24.89,38.73 25.15,38.73 | 26.8,38.73 27.69,38.73 | IC3.8 22.23,36.83 21.84,37.21 21.84,38.35 22.23,38.73 | v8.26,9.02 13.84,9.02 18.8,4.06 25.91,4.06 26.92,5.08 26.92,10.54 29.21,12.83 29.21,14.1 29.84,14.73 35.94,14.73 40.51,19.3 40.51,24.89 41.27,25.65 41.27,28.45 41.91,29.08 48.13,29.08 v48.26,29.21 | C6.1 34.29,38.73 32.13,36.58 32.13,33.27 32.89,32.51 42.04,32.51 42.8,33.27

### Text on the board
Top: dwal1011 / helu1011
